TYPE STR_EL6022 :
STRUCT
	//将EL6022上面的2 3短接，7 8短接
	DATAIN1:ARRAY[0..21] OF USINT;
	DATAIN2:ARRAY[0..21] OF USINT;
	DATAOUT1:ARRAY[0..21] OF USINT;
	DATAOUT2:ARRAY[0..21] OF USINT;
END_STRUCT
END_TYPE
